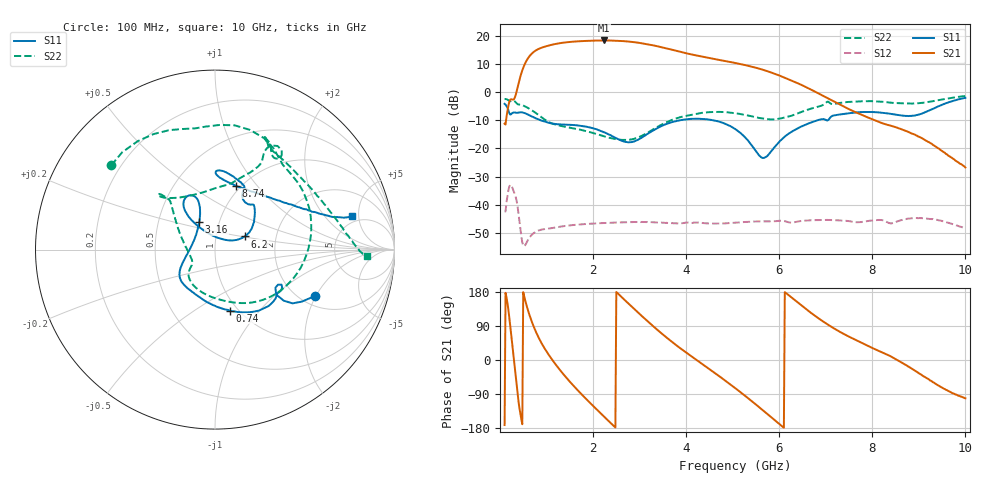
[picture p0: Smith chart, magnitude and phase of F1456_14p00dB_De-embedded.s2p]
! Integrated Device Technology
! Corporate Headquarters
! 6024 Silver Creek Valley Road
! San Jose, CA 95138  USA
! Phone:  1-408-284-8200
! Toll Free:  1-800-223-1366
! Webpage:  http://www.idt.com/
! Timing and RF Division
! 515 Groton Road, Suite 102
! Westford, MA 01886-6024
! Device:  F1456
! Description: 6-bit 0.5 dB Transmit Variable Gain Amplifier
! Frequency:  2100.0 -  2950.00 MHz
! Package:  6x6 mm Thin QFN Plastic Package: 28 pin
! State:  28
! Atten State:  14.0 dB
! Voltage:  +5.00 Volts
! Current:  217.008 mA
! Data:  The device was measured on a the F1455 evaluation board which has
!  individual transmission lines to the RF pins.  Data was collected
!  using a calibrated network analyzer.  The evaluation board was
!  de-embedded using a TRL calibration technique.
!  The reference plane is the edge of the package pin.
!  Pin  1 = CSb
!  Pin  2 = DATA
!  Pin  3 = CLK
!  Pin  4 = RSET
!  Pin  5 = GND
!  Pin  6 = RFIN  = Port 1
!  Pin  7 = GND
!  Pin  8 = NC
!  Pin  9 = NC
!  Pin 10 = NC
!  Pin 11 = NC
!  Pin 12 = NC
!  Pin 13 = NC
!  Pin 14 = /STBY
!  Pin 15 = GND
!  Pin 16 = RFOUT  = Port 2
!  Pin 17 = GND
!  Pin 18 = NC
!  Pin 19 = NC
!  Pin 20 = NC
!  Pin 21 = GND
!  Pin 22 = NC
!  Pin 23 = GND
!  Pin 24 = NC
!  Pin 25 = NC
!  Pin 26 = NC
!  Pin 27 = GND
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# GHz S dB R 50
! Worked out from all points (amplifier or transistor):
!   496 points, 100 MHz to 10 GHz, reference 50 ohm
!   highest |S21| = 18.2 dB at 2.24 GHz (marker M1)
!   |S21| within 3 dB of that: 830.8 MHz to 3.628 GHz (2.797 GHz wide, 125 % of centre)
!   unconditionally stable (mu >= 1): start of sweep to end of sweep
!   at 1.74 GHz: K = 12.63, MAG = 18.5 dB, |S12| = -47.0 dB
!   at 5.06 GHz: K = 25.17, MAG = 11.3 dB, |S12| = -46.4 dB
!   at 10 GHz: K = 318.55, MAG = -17.2 dB, |S12| = -48.4 dB
!   S11 on the Smith chart (normalised r, x): 100 MHz: 2.35, -1.97; 740 MHz: 0.92, -0.71; 3.16 GHz: 0.80, +0.26; 6.2 GHz: 1.38, +0.21; 8.74 GHz: 0.95, +0.79; 10 GHz: 4.23, +4.07
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0.1  -4.24 -25.1  -11.27 -171.7  -42.33 47.5  -2.56 140.9
0.32  -7.29 -32.2  -1.99 -21.3  -36.32 -145.5  -3.37 66.3
0.44  -7.22 -41.9  5.56 -143.2  -48.73 137.1  -4.53 38.4
0.58  -7.85 -58.9  11.35 140.3  -53.14 166.7  -5.48 5.2
0.74  -9.12 -76.3  14.38 83.7  -49.90 135.9  -7.11 -28.5
0.96  -10.54 -97.6  16.04 30.5  -48.65 94.3  -9.81 -66.8
1.18  -11.36 -114.6  16.96 -9.1  -48.12 68.6  -11.53 -93.7
1.48  -11.65 -131.2  17.69 -54.3  -47.35 43.1  -12.61 -119.7
1.76  -12.06 -142.2  18.02 -91.4  -46.93 24.4  -13.53 -133.9
2.24  -14.31 -158.4  18.25 -149.8  -46.49 -2.4  -15.73 -144.7
2.64  -17.46 172.6  18.03 163.0  -46.25 -22.6  -17.03 -156.6
3.16  -14.97 119.4  16.94 103.6  -46.12 -48.5  -14.60 163.8
3.4  -12.67 111.0  16.14 77.7  -46.30 -60.1  -12.28 148.6
3.72  -10.61 109.2  14.88 45.5  -46.60 -74.3  -9.75 136.6
4.08  -9.59 114.0  13.41 12.7  -46.45 -89.2  -8.22 132.8
5.06  -13.22 128.6  10.25 -74.7  -46.37 -131.9  -7.56 135.6
5.66  -23.41 71.2  7.80 -133.8  -45.92 -165.2  -9.49 117.1
6.2  -14.82 23.8  4.44 171.3  -46.24 161.5  -8.72 79.7
6.7  -10.74 40.3  0.68 122.8  -45.52 136.3  -5.86 63.2
8.36  -7.69 88.1  -11.81 11.9  -46.52 65.3  -3.79 62.5
8.74  -8.51 71.8  -13.94 -14.4  -45.00 57.8  -4.10 49.2
10  -2.11 13.7  -26.80 -101.0  -48.42 -25.1  -1.46 -2.5
